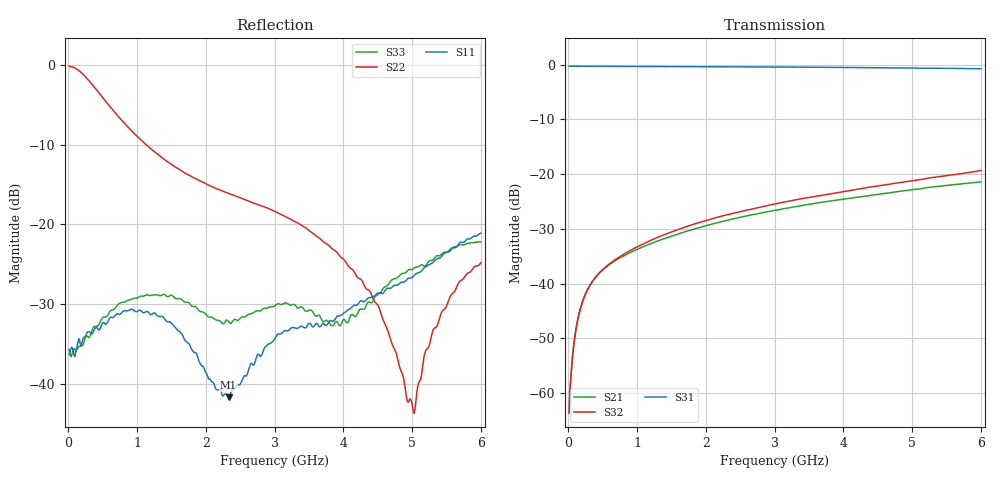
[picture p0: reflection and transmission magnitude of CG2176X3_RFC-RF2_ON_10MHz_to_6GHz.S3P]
!CEL
!CG2176X3
!Port1: RFC Port2: RF1  Port3: RF2
!Freq	S11 S12	S13 S21 S22 S23 S31 S32 S33
# Hz S dB R 50
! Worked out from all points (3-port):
!   600 points, 10 MHz to 6 GHz, reference 50 ohm
!   strongest paths, dB at 10 MHz, 1.51 GHz, 3.01 GHz, 4.51 GHz, 6 GHz:
!     S31: -0.3, -0.4, -0.4, -0.6, -0.7
!     S32: -63.7, -30.5, -25.4, -22.1, -19.3
!     S21: -63.5, -31.3, -26.6, -23.7, -21.4
!   lowest |S11| = -41.6 dB at 2.33 GHz (marker M1), VSWR 1.02, Z = 49.4 + j0.521 ohm
!   |S11| at or under -10 dB: start of sweep to end of sweep
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1e7  -36.30 -1.3  -63.61 47.6  -0.29 -0.2
     -63.51 48.3  -0.19 -1.7  -63.86 48.0
     -0.28 -0.2  -63.72 47.7  -35.66 -5.9
1.5e8  -34.32 10.8  -45.68 73.5  -0.30 -1.5
       -45.68 73.6  -0.73 -20.6  -45.91 75.1
       -0.30 -1.5  -45.86 75.1  -35.29 20.0
4.2e8  -32.99 33.9  -38.48 64.2  -0.31 -4.0
       -38.46 64.1  -3.28 -48.0  -38.48 67.4
       -0.31 -4.0  -38.49 67.6  -32.72 37.2
1.36e9  -31.52 55.4  -31.92 60.9  -0.35 -12.4
        -31.94 60.7  -11.62 -88.2  -31.28 65.6
        -0.35 -12.4  -31.26 65.6  -28.84 36.1
2.33e9  -41.65 140.4  -28.36 59.5  -0.41 -21.0
        -28.38 59.3  -16.11 -107.8  -27.41 63.9
        -0.41 -21.0  -27.37 64.1  -32.18 -14.8
3.01e9  -34.19 -174.4  -26.56 56.5  -0.44 -27.0
        -26.62 56.8  -18.40 -110.6  -25.45 61.7
        -0.44 -27.1  -25.43 61.6  -30.12 -49.2
4.38e9  -29.20 120.6  -23.86 49.7  -0.54 -39.6
        -23.92 49.7  -28.31 -101.1  -22.45 56.4
        -0.54 -39.6  -22.40 56.6  -29.73 -6.2
5.02e9  -26.50 104.6  -22.84 45.3  -0.61 -45.5
        -22.82 45.1  -43.54 -172.6  -21.17 53.1
        -0.62 -45.5  -21.17 53.3  -25.53 -4.9
5.31e9  -24.72 98.7  -22.39 43.7  -0.66 -48.2
        -22.35 43.3  -33.13 133.1  -20.59 51.6
        -0.66 -48.2  -20.61 51.9  -24.36 -8.6
6e9  -21.09 90.0  -21.39 37.5  -0.77 -55.0
     -21.43 38.9  -24.80 126.2  -19.39 47.4
     -0.74 -55.0  -19.33 46.3  -22.19 -10.7
